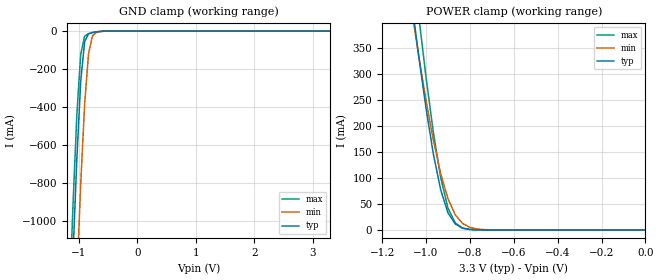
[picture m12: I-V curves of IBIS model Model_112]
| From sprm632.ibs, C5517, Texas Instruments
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| Model based on original model for IC33THYPU
|   Sub model IC33THY_PU_OFF_COM_3P3
[model]   Model_112
|[Description]  [3.3V-INPUT-PU_OFF-X, COM]
|   PU_OFF,COM,
|[Input Load]   PU_OFF
|[Output Drive]
|Voltage   3.3V
|Mode   INPUT
Model_type   Input
Polarity   Non-Inverting
Vinl =  0.8
Vinh =  2
C_comp   0.86952386p  0.83844711p  0.87673039p
[Model Spec]
Vinl   0.8   0.8   0.8
Vinh   2   2   2
[Temperature Range]   25   105   -10
[Voltage Range]   3.3   2.97   3.63
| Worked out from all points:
|   GND clamp passes 1 mA (typ) near -0.59 V on its own axis
|   POWER clamp passes 1 mA (typ) near -0.80 V on its own axis
[POWER_clamp]
-3.3V     9.572A     8.243A     10.62A
-1.067V   445.5mA    428mA      539.5mA
-1.033V   336mA      335.9mA    413.4mA
-1V       234.9mA    250.2mA    294.9mA
-966.7mV  147mA      173.6mA    188.8mA
-933.3mV  77.87mA    109.2mA    101.7mA
-900mV    33.06mA    60.43mA    42.27mA
-866.7mV  11.59mA    29.28mA    13.52mA
-833.3mV  3.563mA    12.55mA    3.583mA
-800mV    1.024mA    4.944mA    867.8uA
-733.3mV  87.24uA    726.8uA    54.46uA
0V        365.2pA    3.923nA    431.9pA
[GND_clamp]
-3.3V     -22.43A    -23.04A    -22.19A
-1.167V   -1.756A    -2.441A    -1.482A
-1.1V     -1.191A    -1.863A    -926.9mA
-1.033V   -674.7mA   -1.312A    -441.8mA
-966.7mV  -263.3mA   -806.2mA   -121.3mA
-900mV    -56.13mA   -384.9mA   -27.09mA
-833.3mV  -14.32mA   -119.2mA   -13.36mA
-766.7mV  -7.053mA   -25.65mA   -8.116mA
-700mV    -3.748mA   -6.724mA   -4.335mA
-633.3mV  -1.654mA   -2.556mA   -1.81mA
3.3V      365.2pA    64.64nA    306.9pA
